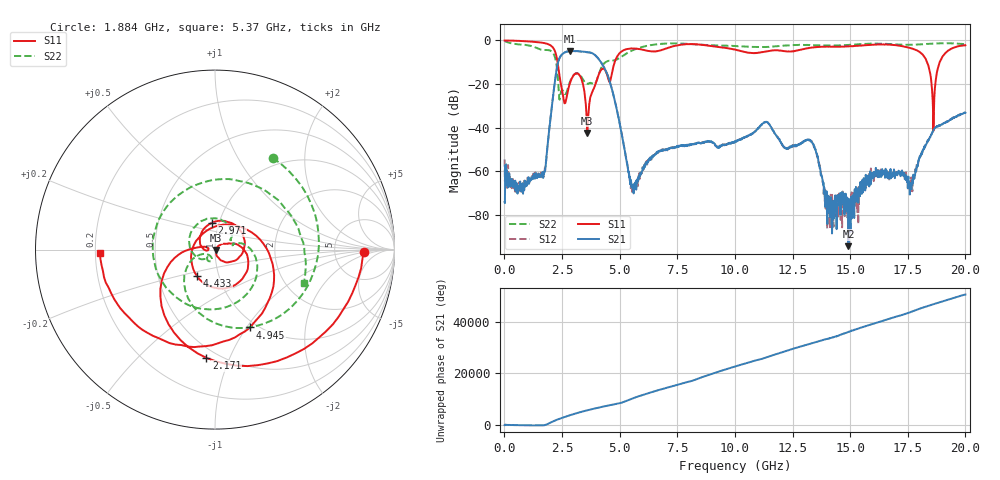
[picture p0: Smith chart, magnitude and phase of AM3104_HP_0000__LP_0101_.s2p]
!Created with skrf (http://scikit-rf.org).
# Hz S RI R 50.0
!freq ReS11 ImS11 ReS21 ImS21 ReS12 ImS12 ReS22 ImS22
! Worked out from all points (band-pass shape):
!   1601 points, 10 MHz to 20 GHz, reference 50 ohm
!   highest |S21| = -4.83 dB at 2.846 GHz (marker M1); lowest = -94.3 dB at 14.93 GHz (marker M2)
!   |S21| within 3 dB of the highest: 2.404 GHz to 4.041 GHz (1.637 GHz wide, 50.8 % of centre)
!   lowest |S11| = -42.4 dB at 3.596 GHz (marker M3), VSWR 1.02, Z = 50.7 - j0.247 ohm
!   |S11| at or under -10 dB: 2.308 GHz to 4.784 GHz (2.477 GHz wide, 69.8 % of centre); 18.34 GHz to 18.88 GHz (542.7 MHz wide, 2.92 % of centre)
!   |S22| runs from -27.1 to -0.2 dB; largest |S21 - S12| = 0.0046
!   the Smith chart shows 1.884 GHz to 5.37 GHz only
!   S11 on the Smith chart (normalised r, x): 1.884 GHz: 11, -1; 2.171 GHz: 0.43, -0.83; 2.971 GHz: 0.92, +0.28; 4.433 GHz: 0.79, -0.24; 4.945 GHz: 0.93, -1.04; 5.37 GHz: 0.22, -0.01
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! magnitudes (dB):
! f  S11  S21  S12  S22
! 10 MHz  0.0  -74.0  -54.5  -0.2
! 772.1 MHz  -0.3  -67.4  -67.3  -1.9
! 1.884 GHz  -1.6  -46.9  -47.0  -4.4
! 2.171 GHz  -4.4  -20.5  -20.5  -7.0
! 2.584 GHz  -27.7  -5.7  -5.7  -24.0
! 2.846 GHz  -19.6  -4.8  -4.9  -18.9
! 2.971 GHz  -16.5  -4.9  -4.9  -16.3
! 3.346 GHz  -17.7  -5.1  -5.1  -16.7
! 3.596 GHz  -42.4  -5.4  -5.4  -19.9
! 4.433 GHz  -15.0  -14.8  -14.8  -9.7
! 4.945 GHz  -6.4  -35.0  -35.0  -8.4
! 5.37 GHz  -3.9  -59.7  -59.3  -5.6
! 6.682 GHz  -4.8  -51.0  -50.8  -1.7
! 10.01 GHz  -4.2  -46.6  -46.3  -2.5
! 13.34 GHz  -3.2  -46.7  -46.2  -2.2
! 14.03 GHz  -2.8  -73.7  -76.3  -2.3
! 14.93 GHz  -2.7  -94.3  -75.9  -2.0
! 16.68 GHz  -1.9  -61.8  -62.0  -1.6
! 17.64 GHz  -3.6  -66.2  -66.0  -2.0
! 18.61 GHz  -41.4  -41.2  -41.1  -1.4
! 19.01 GHz  -7.3  -38.3  -38.3  -1.3
! 20 GHz  -2.2  -33.1  -33.2  -1.7
